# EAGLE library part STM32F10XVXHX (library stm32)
ST STM32F 100 pin BGA
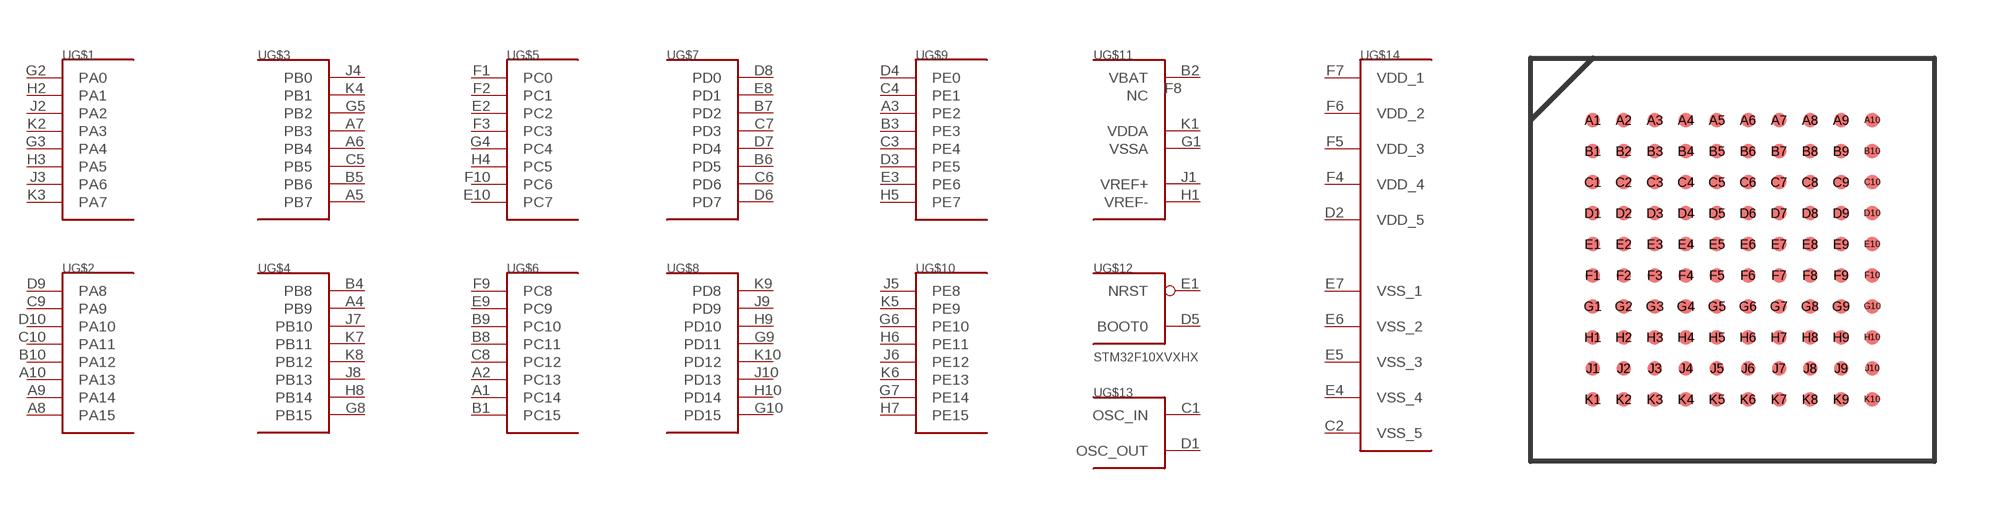
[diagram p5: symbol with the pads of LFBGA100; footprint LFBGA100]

Designator prefix U; gates G$1=PORT_A_L G$2=PORT_A_H G$3=PORT_B_L G$4=PORT_B_H G$5=PORT_C_L G$6=PORT_C_H G$7=PORT_D_L G$8=PORT_D_H G$9=PORT_E_L G$10=PORT_E_H G$11=BAT_AN_L G$12=BOOT_RST G$13=OSC G$14=VCC_VSS_L

## STM32F10XVXHX  [LFBGA100]
A1  G$6:PC14
A2  G$6:PC13
A3  G$9:PE2
A4  G$4:PB9
A5  G$3:PB7
A6  G$3:PB4
A7  G$3:PB3
A8  G$2:PA15
A9  G$2:PA14
A10  G$2:PA13
B1  G$6:PC15
B2  G$11:VBAT  pwr
B3  G$9:PE3
B4  G$4:PB8
B5  G$3:PB6
B6  G$7:PD5
B7  G$7:PD2
B8  G$6:PC11
B9  G$6:PC10
B10  G$2:PA12
C1  G$13:OSC_IN  in
C2  G$14:VSS_5  pwr
C3  G$9:PE4
C4  G$9:PE1
C5  G$3:PB5
C6  G$7:PD6
C7  G$7:PD3
C8  G$6:PC12
C9  G$2:PA9
C10  G$2:PA11
D1  G$13:OSC_OUT  out
D2  G$14:VDD_5  pwr
D3  G$9:PE5
D4  G$9:PE0
D5  G$12:BOOT0  in
D6  G$7:PD7
D7  G$7:PD4
D8  G$7:PD0
D9  G$2:PA8
D10  G$2:PA10
E1  G$12:NRST  in
E2  G$5:PC2
E3  G$9:PE6
E4  G$14:VSS_4  pwr
E5  G$14:VSS_3  pwr
E6  G$14:VSS_2  pwr
E7  G$14:VSS_1  pwr
E8  G$7:PD1
E9  G$6:PC9
E10  G$5:PC7
F1  G$5:PC0
F2  G$5:PC1
F3  G$5:PC3
F4  G$14:VDD_4  pwr
F5  G$14:VDD_3  pwr
F6  G$14:VDD_2  pwr
F7  G$14:VDD_1  pwr
F8  G$11:NC  nc
F9  G$6:PC8
F10  G$5:PC6
G1  G$11:VSSA  pwr
G2  G$1:PA0
G3  G$1:PA4
G4  G$5:PC4
G5  G$3:PB2
G6  G$10:PE10
G7  G$10:PE14
G8  G$4:PB15
G9  G$8:PD11
G10  G$8:PD15
H1  G$11:VREF-  in
H2  G$1:PA1
H3  G$1:PA5
H4  G$5:PC5
H5  G$9:PE7
H6  G$10:PE11
H7  G$10:PE15
H8  G$4:PB14
H9  G$8:PD10
H10  G$8:PD14
J1  G$11:VREF+  in
J2  G$1:PA2
J3  G$1:PA6
J4  G$3:PB0
J5  G$10:PE8
J6  G$10:PE12
J7  G$4:PB10
J8  G$4:PB13
J9  G$8:PD9
J10  G$8:PD13
K1  G$11:VDDA  pwr
K2  G$1:PA3
K3  G$1:PA7
K4  G$3:PB1
K5  G$10:PE9
K6  G$10:PE13
K7  G$4:PB11
K8  G$4:PB12
K9  G$8:PD8
K10  G$8:PD12

## Footprint LFBGA100 (pad centres in mm)
LFBGA100 0.8mm pictch bga
smd 0.37 x 0.37: A1 0,7.2; A2 0.8,7.2; A3 1.6,7.2; A4 2.4,7.2; A5 3.2,7.2; A6 4,7.2; A7 4.8,7.2; A8 5.6,7.2; A9 6.4,7.2; A10 7.2,7.2; B1 0,6.4; B2 0.8,6.4; B3 1.6,6.4; B4 2.4,6.4; B5 3.2,6.4; B6 4,6.4; B7 4.8,6.4; B8 5.6,6.4; B9 6.4,6.4; B10 7.2,6.4; C1 0,5.6; C2 0.8,5.6; C3 1.6,5.6; C4 2.4,5.6; C5 3.2,5.6; C6 4,5.6; C7 4.8,5.6; C8 5.6,5.6; C9 6.4,5.6; C10 7.2,5.6; D1 0,4.8; D2 0.8,4.8; D3 1.6,4.8; D4 2.4,4.8; D5 3.2,4.8; D6 4,4.8; D7 4.8,4.8; D8 5.6,4.8; D9 6.4,4.8; D10 7.2,4.8; E1 0,4; E2 0.8,4; E3 1.6,4; E4 2.4,4; E5 3.2,4; E6 4,4; E7 4.8,4; E8 5.6,4; E9 6.4,4; E10 7.2,4; F1 0,3.2; F2 0.8,3.2; F3 1.6,3.2; F4 2.4,3.2; F5 3.2,3.2; F6 4,3.2; F7 4.8,3.2; F8 5.6,3.2; F9 6.4,3.2; F10 7.2,3.2; G1 0,2.4; G2 0.8,2.4; G3 1.6,2.4; G4 2.4,2.4; G5 3.2,2.4; G6 4,2.4; G7 4.8,2.4; G8 5.6,2.4; G9 6.4,2.4; G10 7.2,2.4; H1 0,1.6; H2 0.8,1.6; H3 1.6,1.6; H4 2.4,1.6; H5 3.2,1.6; H6 4,1.6; H7 4.8,1.6; H8 5.6,1.6; H9 6.4,1.6; H10 7.2,1.6; J1 0,0.8; J2 0.8,0.8; J3 1.6,0.8; J4 2.4,0.8; J5 3.2,0.8; J6 4,0.8; J7 4.8,0.8; J8 5.6,0.8; J9 6.4,0.8; J10 7.2,0.8; K1 0,0; K2 0.8,0; K3 1.6,0; K4 2.4,0; K5 3.2,0; K6 4,0; K7 4.8,0; K8 5.6,0; K9 6.4,0; K10 7.2,0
